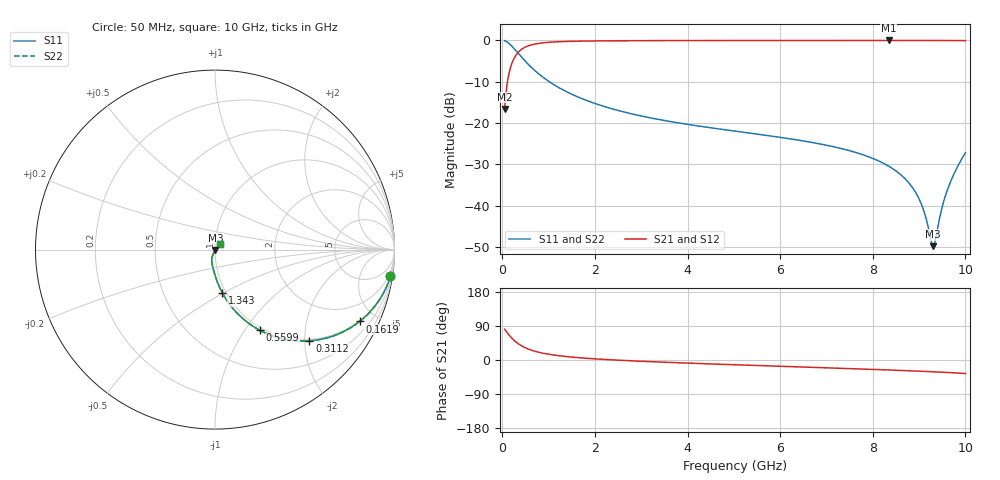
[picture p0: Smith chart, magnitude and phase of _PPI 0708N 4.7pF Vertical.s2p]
! S-Parameter data specifications (vertical orientation):
! Substrate: 40-mil Rogers 3003C, Substrate thickness, H=1.016mm, Dielectric constant, Er=3, Conductor thickness, T_mtl=0.043mm, Loss Tangent, Tand=0.003
! PCB Mounting Pad Footprint: Pad width, PadW=2.54mm , Pad length, PadL=0.51mm , Pad gap, PadG (edge-to-edge)=0.71mm , Reference planes=1.73mm apart
! Created Tue Jan 16 08:45:37 2018
# GHz S MA R 50
! 2 Port Network Data from SP1.SP block
! freq  magS11  angS11  magS21  angS21  magS12  angS12  magS22  angS22
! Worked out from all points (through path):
!   801 points, 50 MHz to 10 GHz, reference 50 ohm
!   highest |S21| = -0.03 dB at 8.346 GHz (marker M1); lowest = -16.6 dB at 50 MHz (marker M2)
!   group delay of S21, straight-line fit = 17.2 ps
!   lowest |S11| = -49.8 dB at 9.303 GHz (marker M3), VSWR 1.01, Z = 50.3 - j0.186 ohm
!   |S11| at or under -10 dB: 1.014 GHz to end of sweep
!   |S22| runs from -49.8 to -0.1 dB; largest |S21 - S12| = 0
!   S11 on the Smith chart (normalised r, x): 50 MHz: 1, -13; 161.9 MHz: 0.96, -4.04; 311.2 MHz: 0.96, -2.10; 559.9 MHz: 0.96, -1.17; 1.343 GHz: 0.96, -0.50; 10 GHz: 1.06, +0.07
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0.05  0.9889 -8.7  0.1482 81.3  0.1482 81.3  0.9889 -8.7
0.1619375  0.8996 -26.4  0.4365 63.5  0.4365 63.5  0.8996 -26.4
0.3111875  0.7316 -44.0  0.6814 45.9  0.6814 45.9  0.7316 -44.0
0.5599375  0.5132 -61.0  0.8578 28.9  0.8578 28.9  0.5132 -61.0
0.870875  0.3606 -71.8  0.9322 18.1  0.9322 18.1  0.3606 -71.8
1.3435  0.2461 -80.3  0.9686 9.6  0.9686 9.6  0.2461 -80.3
1.716625  0.1974 -84.3  0.9796 5.5  0.9796 5.5  0.1974 -84.3
3.370812  0.1104 -94.8  0.9928 -5.3  0.9928 -5.3  0.1104 -94.8
5.025  0.07968 -101.8  0.9954 -12.6  0.9954 -12.6  0.07968 -101.8
6.691625  0.05806 -107.9  0.9965 -19.4  0.9965 -19.4  0.05806 -107.9
7.674188  0.04326 -111.0  0.997 -23.4  0.997 -23.4  0.04326 -111.0
8.345812  0.02996 -112.3  0.9971 -26.3  0.9971 -26.3  0.02996 -112.3
8.681625  0.02158 -111.5  0.997 -27.9  0.997 -27.9  0.02158 -111.5
8.930375  0.01429 -108.4  0.9969 -29.1  0.9969 -29.1  0.01429 -108.4
9.092063  0.008991 -101.4  0.9967 -29.9  0.9967 -29.9  0.008991 -101.4
9.25375  0.003883 -67.2  0.9965 -30.8  0.9965 -30.8  0.003883 -67.2
9.3035  0.003229 -35.0  0.9964 -31.0  0.9964 -31.0  0.003229 -35.0
9.35325  0.003854 -1.0  0.9963 -31.3  0.9963 -31.3  0.003854 -1.0
9.490063  0.009202 34.5  0.9959 -32.1  0.9959 -32.1  0.009202 34.5
9.614437  0.01567 42.2  0.9955 -32.9  0.9955 -32.9  0.01567 42.2
9.801  0.02745 45.8  0.9944 -34.2  0.9944 -34.2  0.02745 45.8
10  0.04355 46.3  0.9926 -35.7  0.9926 -35.7  0.04355 46.3
